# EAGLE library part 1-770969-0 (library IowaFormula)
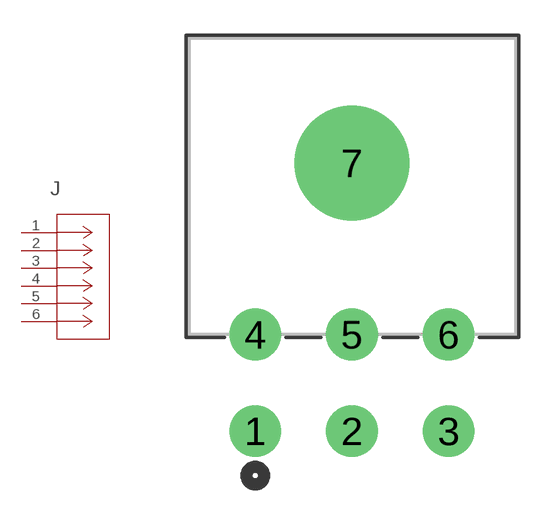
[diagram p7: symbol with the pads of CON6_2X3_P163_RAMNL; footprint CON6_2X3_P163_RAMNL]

Designator prefix J

## 1-770969-0 (MANUFACTURER_PART_NUMBER: 17709690; VENDOR: TE Connectivity)  [CON6_2X3_P163_RAMNL]
1  1  pas
2  2  pas
3  3  pas
4  4  pas
5  5  pas
6  6  pas

## Footprint CON6_2X3_P163_RAMNL (pad centres in mm)
drill 1.473 pad 1.981: 1 -8.28,-4.14; 2 -4.14,-4.14; 3 0,-4.14; 4 -8.28,0; 5 -4.14,0; 6 0,0
drill 3.912 pad 3.912: 7 -4.14,7.341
